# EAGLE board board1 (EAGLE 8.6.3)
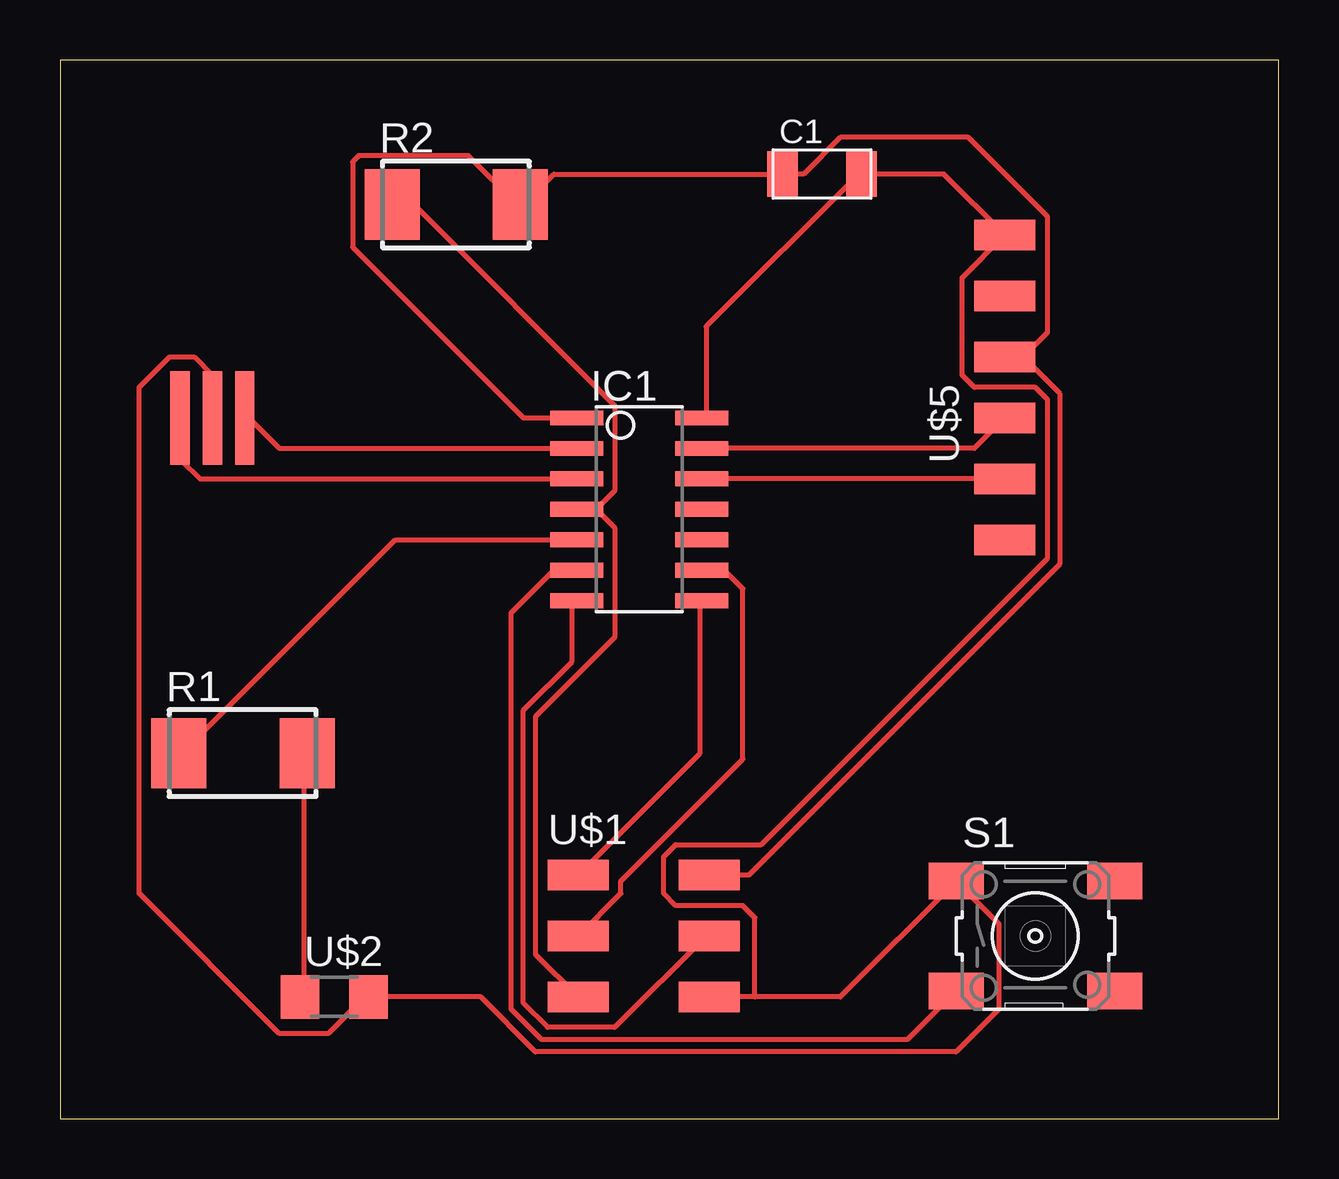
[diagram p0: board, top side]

Size 50.78 x 44.12 mm. Coordinates in mm from the lower left corner, seen from the top.
Outline: 0,0 50.78,0 50.78,44.12 0,44.12 0,0
Copper layers (1*16): Top 0.035mm / dielectric 1.5mm / Bottom 0.035mm
Design rules "default *": minimum track width 8mil, minimum drill 0.35mm, track to track 12mil, track to pad 12mil, pad to pad 6mil, via to via 6mil, smd to smd 6mil, copper to edge 40mil, drill to drill 6mil, minimum pad ring 10mil, minimum via ring 8mil, stop-mask expansion 4mil, vias tented up to drill 0mil, thermal gap 10mil

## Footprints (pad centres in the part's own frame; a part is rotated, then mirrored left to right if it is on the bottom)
C1206FAB = smd 1.27 x 1.905: 1 -1.651,0; 2 1.651,0
SOIC14 = smd 0.61 x 2.21: 1 -3.81,-2.603; 2 -2.54,-2.603; 3 -1.27,-2.603; 4 0,-2.603; 5 1.27,-2.603; 6 2.54,-2.603; 7 3.81,-2.603; 8 3.81,2.603; 9 2.54,2.603; 10 1.27,2.603; 11 0,2.603; 12 -1.27,2.603; 13 -2.54,2.603; 14 -3.81,2.603
WSC2515 = smd 2.29 x 2.92: 1 -2.675,0; 2 2.675,0
6MM_SWITCH = smd 2.286 x 1.524: 1 -3.302,2.286; 2 3.302,2.286; 3 -3.302,-2.286; 4 3.302,-2.286
2X03SMD = smd 2.54 x 1.27: 1 -2.54,2.54; 2 2.92,2.54; 3 -2.54,0; 4 2.92,0; 5 -2.54,-2.54; 6 2.92,-2.54
LED1206 = smd 1.6 x 1.803: 1 -1.422,0; 2 1.422,0
1X06SMD = smd 2.54 x 1.27: 1 0,6.35; 2 0,3.81; 3 0,1.27; 4 0,-1.27; 5 0,-3.81; 6 0,-6.35
EFOBM = smd 0.8 x 3.9: 1 -1.35,0; 2 0,0; 3 1.35,0

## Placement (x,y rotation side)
C1  1uf  [C1206FAB]  31.75,39.37 0 top
IC1  ATTINY44-SSU  [SOIC14]  24.13,25.4 270 top
R1  499k  [WSC2515]  7.62,15.24 0 top
R2  10k  [WSC2515]  16.51,38.1 0 top
S1  1  [6MM_SWITCH]  40.64,7.62 0 top
U$1  AVRISPSMD  [2X03SMD]  24.13,7.62 0 top
U$2  LED  [LED1206]  11.43,5.08 0 top
U$5  FTDI-SMD-HEADER  [1X06SMD]  39.37,30.48 0 top
U$6  RESONATOR  [EFOBM]  6.35,29.21 0 top

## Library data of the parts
C1 IC1 S1 U$1 U$2 U$5 U$6 = fab
R1 R2 = resistor

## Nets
BTN: IC1.6 S1.3
GND: C1.2 IC1.14 S1.1 U$1.6 U$2.2 U$5.1 U$6.2
LED: IC1.5 R1.1
MISO: IC1.8 U$1.1
MOSI: IC1.7 U$1.4
N$2: R1.2 U$2.1
RES01: IC1.3 U$6.1
RES02: IC1.2 U$6.3
RESET: IC1.4 R2.1 U$1.5
RX: IC1.12 U$5.5
SCK: IC1.9 U$1.3
TX: IC1.13 U$5.4
VCC: C1.1 IC1.1 R2.2 U$1.2 U$5.3

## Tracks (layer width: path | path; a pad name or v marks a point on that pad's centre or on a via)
BTN
  Top 0.203: IC1.6 20.57,22.86 18.8,21.08 18.8,4.57 20.07,3.3 35.31,3.3 S1.3
GND
  Top 0.203: IC1.14 26.92,29.21 26.92,33.02 33.27,39.37 C1.2 36.83,39.37 U$5.1 37.59,35.05 37.59,30.99 38.1,30.48 40.64,30.48 41.15,29.97 41.15,23.37 29.21,11.43 25.65,11.43 25.15,10.92 25.15,9.4 25.65,8.89 28.45,8.89 28.96,8.38 28.96,5.08 | 28.96,5.08 32.51,5.08 S1.1 39.12,8.13 39.12,4.57 37.34,2.79 19.81,2.79 17.53,5.08 U$2.2 12.7,5.08 11.18,3.56 9.14,3.56 3.3,9.4 3.3,30.48 4.57,31.75 5.59,31.75 6.35,30.99 U$6.2 | 28.96,5.08 U$1.6
LED
  Top 0.203: IC1.5 13.97,24.13 5.08,15.24 R1.1
MISO
  Top 0.203: U$1.1 26.67,15.24 26.67,21.59 IC1.8
MOSI
  Top 0.203: IC1.7 21.34,21.59 21.34,19.05 19.3,17.02 19.3,4.83 20.32,3.81 23.11,3.81 26.92,7.62 U$1.4
N$2
  Top 0.203: U$2.1 10.16,5.08 10.16,15.24 R1.2
RES01
  Top 0.203: IC1.3 5.84,26.67 5.08,27.43 5.08,29.21 U$6.1
RES02
  Top 0.203: IC1.2 9.14,27.94 7.87,29.21 U$6.3
RESET
  Top 0.203: 22.35,25.4 IC1.4 21.59,25.4 | 22.35,25.4 23.11,26.16 23.11,29.72 14.73,38.1 R2.1 | U$1.5 19.81,6.86 19.81,16.76 23.11,20.07 23.11,24.64 22.35,25.4
RX
  Top 0.203: U$5.5 IC1.12
SCK
  Top 0.203: IC1.9 27.69,22.86 28.45,22.1 28.45,14.99 23.37,9.91 23.37,9.4 U$1.3
TX
  Top 0.203: IC1.13 38.1,27.94 U$5.4
VCC
  Top 0.203: IC1.1 19.3,29.21 12.19,36.32 12.19,39.88 12.45,40.13 17.02,40.13 19.05,38.1 R2.2 19.3,38.1 20.57,39.37 C1.1 30.99,39.37 32.51,40.89 37.85,40.89 41.15,37.59 41.15,32.77 40.13,31.75 | U$1.2 28.7,10.16 41.66,23.11 41.66,30.23 40.13,31.75 | 40.13,31.75 U$5.3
